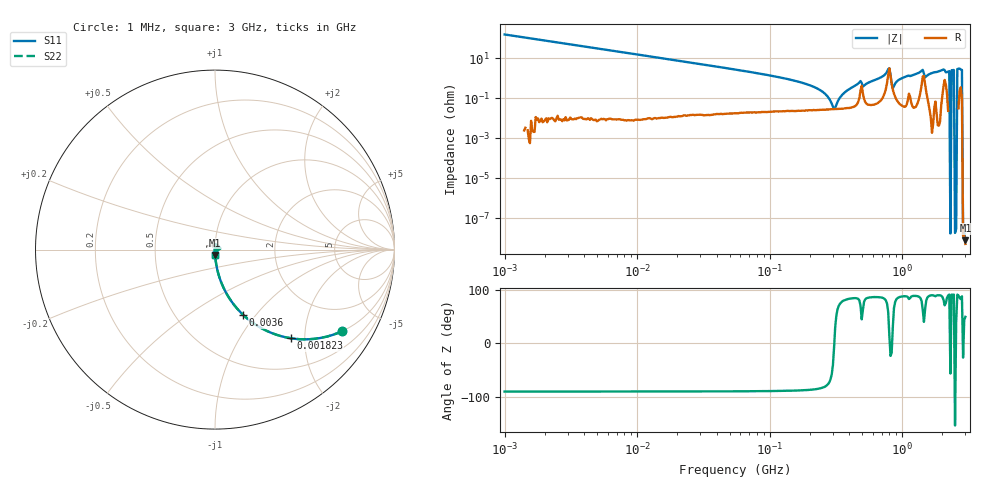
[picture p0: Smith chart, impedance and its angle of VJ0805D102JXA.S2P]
! VJ0805D102JXA
! DATE
! CORRECTED  DATA
# Hz  S  MA  R  50
!Freq	S11M	S11A	S21M	S21A	S12M	S12A	S22M	S22A
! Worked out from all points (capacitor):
!   401 points, 1 MHz to 3 GHz, reference 50 ohm
!   read as one part in series: C = 1.02 nF near 1.041 MHz
!   lowest |Z| = 7.93 nohm at 3 GHz (marker M1)
!   series resonance near 307.4 MHz, so ESL is about 260 pH
!   S11 on the Smith chart (normalised r, x): 1 MHz: 1.00, -3.11; 1.823 MHz: 1.00, -1.71; 3.6 MHz: 1.00, -0.86; 3 GHz: 1.00, -0.06
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1000000  0.8413 -32.7  0.5407 57.3  0.5407 57.3  0.8413 -32.7
1822989  0.6492 -49.5  0.7606 40.5  0.7606 40.5  0.6492 -49.5
3600306  0.3967 -66.6  0.9179 23.4  0.9179 23.4  0.3967 -66.6
3823119  0.3769 -67.8  0.9262 22.1  0.9262 22.1  0.3769 -67.8
1.461624e7  0.1056 -83.9  0.9943 6.1  0.9943 6.1  0.1056 -83.9
5.587962e7  0.02688 -88.1  0.9995 1.5  0.9995 1.5  0.02688 -88.1
1.321429e8  0.009599 -88.1  0.9997 0.5  0.9997 0.5  0.009599 -88.1
2.094008e8  0.004014 -86.2  0.9997 0.2  0.9997 0.2  0.004014 -86.2
2.609752e8  0.001708 -80.9  0.9997 0.1  0.9997 0.1  0.001708 -80.9
3.062963e8  0.0002911 -7.7  0.9997 0.0  0.9997 0.0  0.0002911 -7.7
3.667557e8  0.001906 80.5  0.9997 -0.1  0.9997 -0.1  0.001906 80.5
4.66327e8  0.005475 82.7  0.9993 -0.3  0.9993 -0.3  0.005475 82.7
5.258324e8  0.004829 81.9  0.9993 -0.3  0.9993 -0.3  0.004829 81.9
6.958997e8  0.01135 85.2  0.9991 -0.6  0.9991 -0.6  0.01135 85.2
7.691493e8  0.02112 73.0  0.994 -1.2  0.994 -1.2  0.02112 73.0
8.005644e8  0.03098 13.3  0.9699 -0.4  0.9699 -0.4  0.03098 13.3
8.672962e8  0.004121 65.6  0.9983 -0.2  0.9983 -0.2  0.004121 65.6
9.779672e8  0.009532 86.6  0.9995 -0.5  0.9995 -0.5  0.009532 86.6
1.374365e9  0.02123 83.3  0.9978 -1.2  0.9978 -1.2  0.02123 83.3
1.54974e9  0.01409 84.9  0.9988 -0.8  0.9988 -0.8  0.01409 84.9
2.01032e9  0.02602 85.5  0.9983 -1.5  0.9983 -1.5  0.02602 85.5
3e9  0.02922 -87.3  1.002 -1.7  1.002 -1.7  0.02922 -87.3
